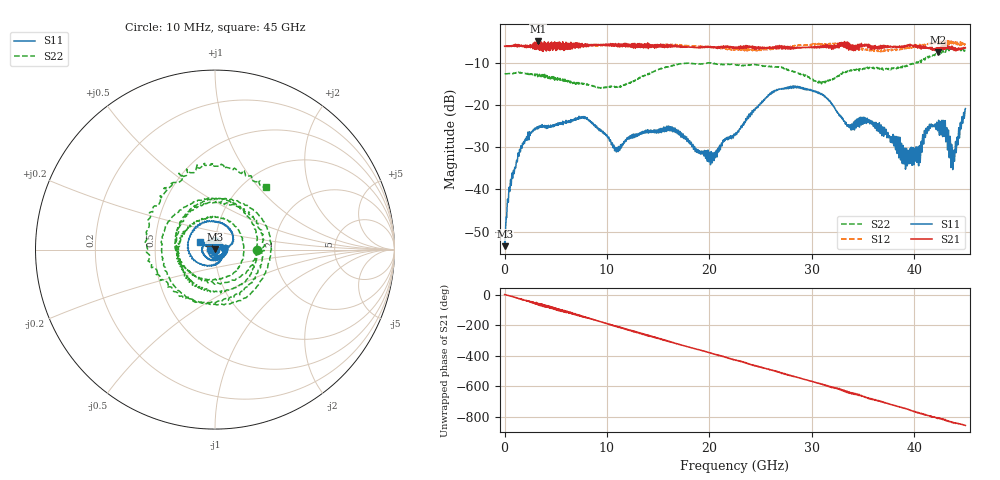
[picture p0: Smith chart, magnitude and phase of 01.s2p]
! 9/19/2025 2:49:21 PM
! C:\USERS\VECTORSTARUSER\DESKTOP\1942\01.S2P
! CHANNEL.1
! TR.MEASUREMENT
! CORRECTED.DATA
! RF.CORRECTION: FULL.TWO.PORT.CAL.PORT.1.2
! AVERAGING.OFF
! IF.BANDWIDTH: 1KHZ
! SWEEPTYPE:  FREQ.SWEEP(Linear)
! Reference Plane Port Info
! PORT:  PORT1  PORT2
! DISTANCE:  0  m  0  m
! TIME:  0  s  0  s
! PHASE.OFFSET:  0 °  0 °
! LOSS:  0  dB  0  dB
! REF.LOSS:  0  dB  0  dB
! REF.FREQ:  0  Hz  0  Hz
! Power Info
! POWER:  -10  dBm  -10  dBm
! EFF.POWER:  -10  dBm  -10  dBm
! SOURCE.ATTEN:  0  dB  0  dB
! TEST.ATTEN:  0  dB  0  dB
# GHZ S RI R 50.0
! FREQ.GHZ  S11RE  S11IM  S21RE  S21IM  S12RE  S12IM  S22RE  S22IM
!; PortSelection: Port_12
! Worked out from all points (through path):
!   1601 points, 10 MHz to 45 GHz, reference 50 ohm
!   highest |S21| = -4.76 dB at 3.272 GHz (marker M1); lowest = -7.4 dB at 42.3 GHz (marker M2)
!   group delay of S21, straight-line fit = 53 ps
!   lowest |S11| = -53.5 dB at 38.12 MHz (marker M3), VSWR 1.00, Z = 49.8 + j0.123 ohm
!   |S11| at or under -10 dB: start of sweep to end of sweep
!   |S22| runs from -15.9 to -6.3 dB; largest |S21 - S12| = 0.14
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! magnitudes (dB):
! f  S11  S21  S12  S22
! 10 MHz  -52.6  -6.0  -6.0  -12.6
! 38.12 MHz  -53.5  -6.0  -6.0  -12.5
! 516.1 MHz  -40.5  -6.1  -6.0  -12.5
! 1.388 GHz  -32.1  -5.9  -5.9  -12.2
! 3.272 GHz  -25.1  -4.8  -6.0  -12.7
! 7.518 GHz  -23.0  -6.0  -5.8  -14.9
! 10.95 GHz  -30.9  -6.0  -5.8  -15.6
! 15.03 GHz  -26.1  -5.8  -5.6  -11.6
! 16.57 GHz  -26.3  -6.1  -5.7  -10.5
! 20.11 GHz  -34.1  -6.0  -6.1  -10.0
! 22.5 GHz  -27.2  -6.3  -6.8  -10.4
! 26.27 GHz  -16.6  -6.5  -6.7  -10.9
! 30.01 GHz  -16.4  -6.1  -5.7  -13.9
! 33.64 GHz  -25.2  -6.4  -5.7  -11.6
! 35.41 GHz  -23.1  -5.6  -6.6  -11.0
! 37.52 GHz  -27.8  -5.9  -6.8  -11.5
! 39.35 GHz  -33.7  -6.0  -6.4  -10.7
! 41.51 GHz  -24.6  -6.2  -5.6  -8.4
! 42.3 GHz  -26.1  -7.4  -5.3  -7.7
! 42.95 GHz  -27.4  -6.5  -5.5  -7.1
! 43.79 GHz  -33.9  -6.7  -4.9  -6.4
! 45 GHz  -20.8  -6.4  -5.6  -7.0
